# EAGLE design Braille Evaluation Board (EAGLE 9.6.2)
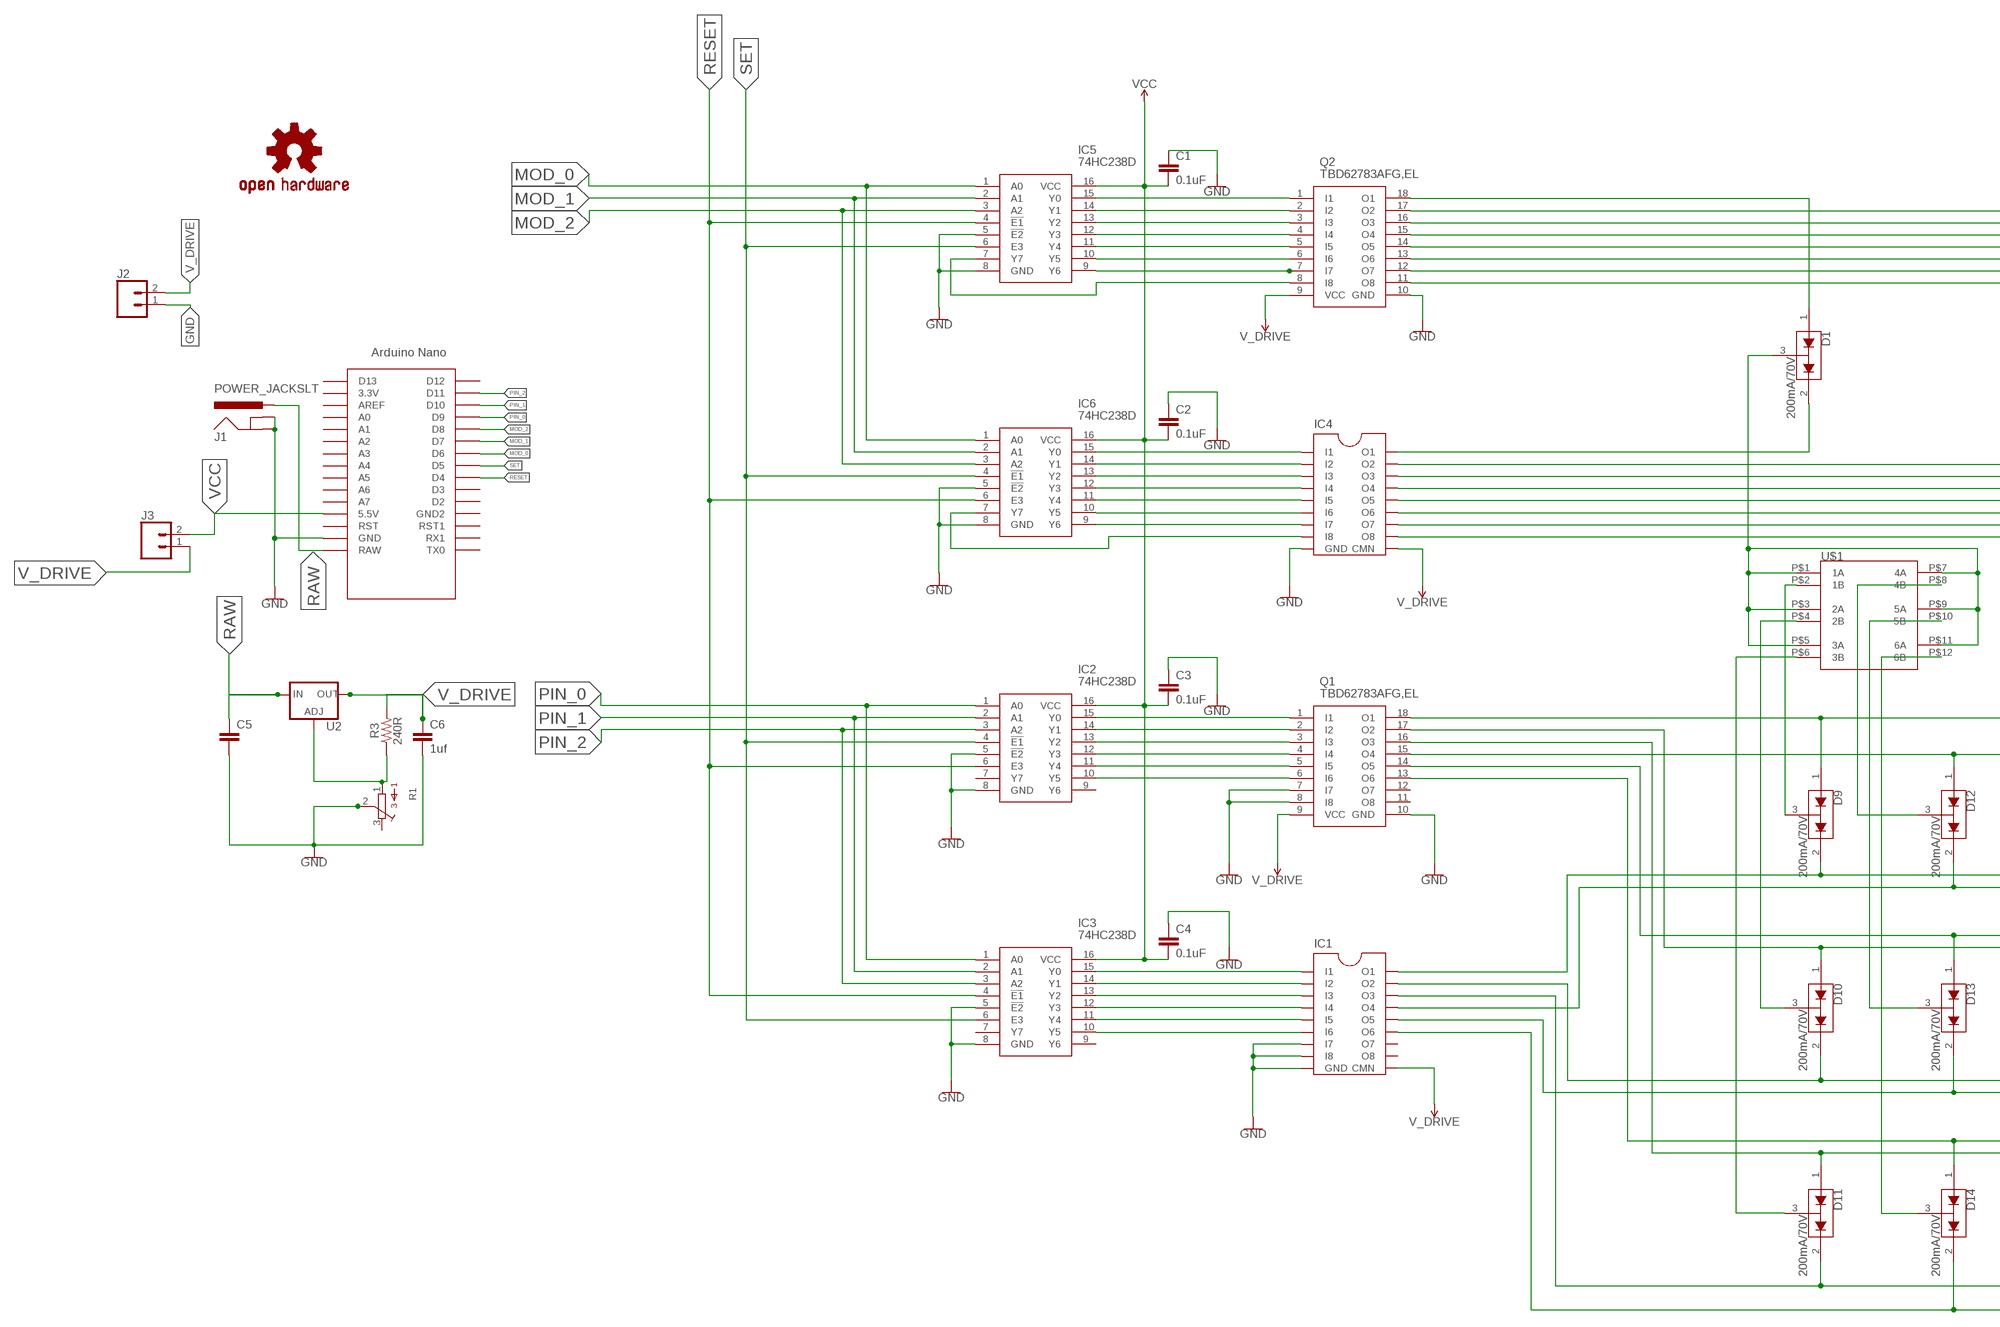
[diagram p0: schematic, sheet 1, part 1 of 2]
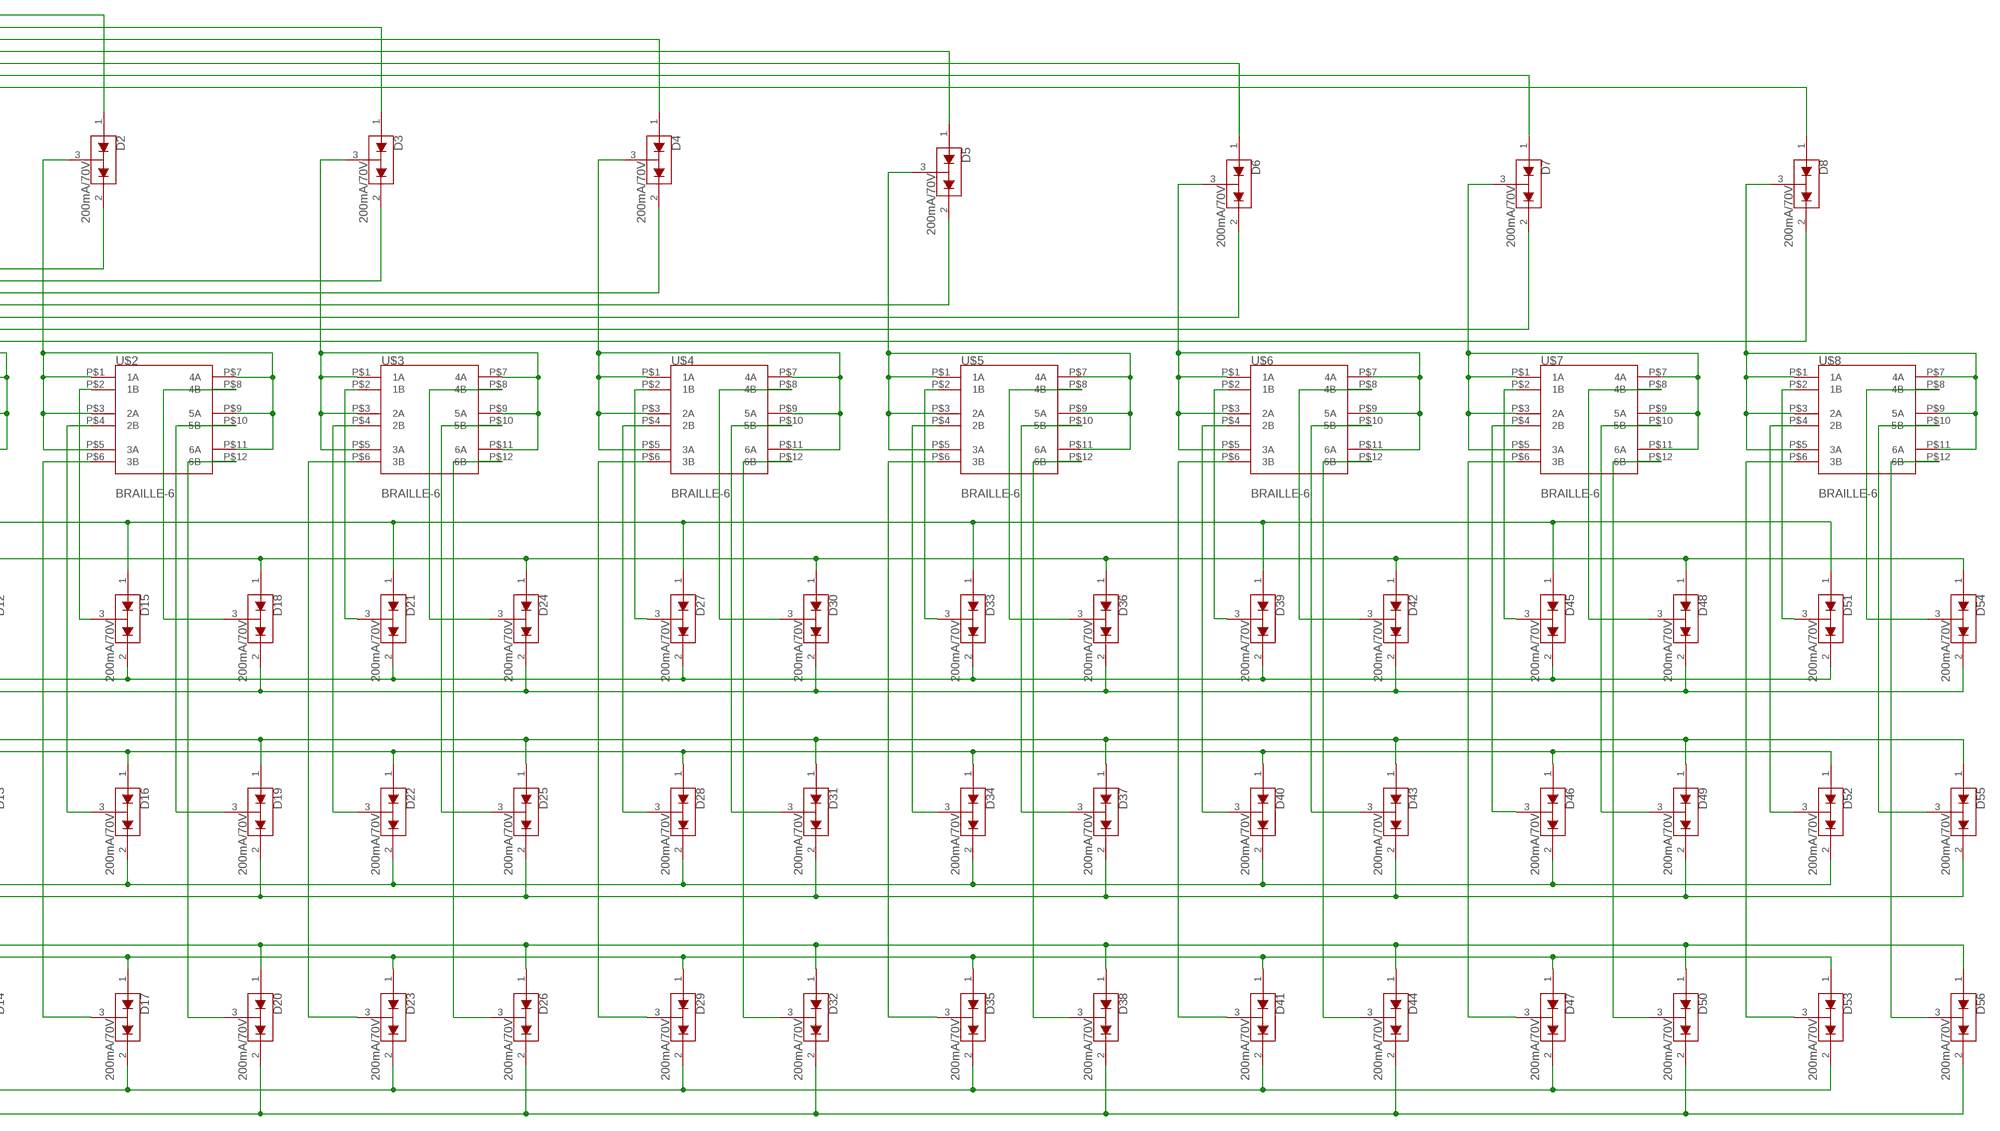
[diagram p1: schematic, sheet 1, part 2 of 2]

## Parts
C1  0.1uF  0.1UF-0603-25V-(+80/-20%)  [0603]
C2  0.1uF  0.1UF-0603-25V-(+80/-20%)  [0603]
C3  0.1uF  0.1UF-0603-25V-(+80/-20%)  [0603]
C4  0.1uF  0.1UF-0603-25V-(+80/-20%)  [0603]
C5  0.1uF  9.0PF-0603-50V-10%  [0603]
C6  1uf  9.0PF-0603-50V-10%  [0603]
D1  200mA/70V  BAV99  [SOT23-3]
D2  200mA/70V  BAV99  [SOT23-3]
D3  200mA/70V  BAV99  [SOT23-3]
D4  200mA/70V  BAV99  [SOT23-3]
D5  200mA/70V  BAV99  [SOT23-3]
D6  200mA/70V  BAV99  [SOT23-3]
D7  200mA/70V  BAV99  [SOT23-3]
D8  200mA/70V  BAV99  [SOT23-3]
D9  200mA/70V  BAV99  [SOT23-3]
D10  200mA/70V  BAV99  [SOT23-3]
D11  200mA/70V  BAV99  [SOT23-3]
D12  200mA/70V  BAV99  [SOT23-3]
D13  200mA/70V  BAV99  [SOT23-3]
D14  200mA/70V  BAV99  [SOT23-3]
D15  200mA/70V  BAV99  [SOT23-3]
D16  200mA/70V  BAV99  [SOT23-3]
D17  200mA/70V  BAV99  [SOT23-3]
D18  200mA/70V  BAV99  [SOT23-3]
D19  200mA/70V  BAV99  [SOT23-3]
D20  200mA/70V  BAV99  [SOT23-3]
D21  200mA/70V  BAV99  [SOT23-3]
D22  200mA/70V  BAV99  [SOT23-3]
D23  200mA/70V  BAV99  [SOT23-3]
D24  200mA/70V  BAV99  [SOT23-3]
D25  200mA/70V  BAV99  [SOT23-3]
D26  200mA/70V  BAV99  [SOT23-3]
D27  200mA/70V  BAV99  [SOT23-3]
D28  200mA/70V  BAV99  [SOT23-3]
D29  200mA/70V  BAV99  [SOT23-3]
D30  200mA/70V  BAV99  [SOT23-3]
D31  200mA/70V  BAV99  [SOT23-3]
D32  200mA/70V  BAV99  [SOT23-3]
D33  200mA/70V  BAV99  [SOT23-3]
D34  200mA/70V  BAV99  [SOT23-3]
D35  200mA/70V  BAV99  [SOT23-3]
D36  200mA/70V  BAV99  [SOT23-3]
D37  200mA/70V  BAV99  [SOT23-3]
D38  200mA/70V  BAV99  [SOT23-3]
D39  200mA/70V  BAV99  [SOT23-3]
D40  200mA/70V  BAV99  [SOT23-3]
D41  200mA/70V  BAV99  [SOT23-3]
D42  200mA/70V  BAV99  [SOT23-3]
D43  200mA/70V  BAV99  [SOT23-3]
D44  200mA/70V  BAV99  [SOT23-3]
D45  200mA/70V  BAV99  [SOT23-3]
D46  200mA/70V  BAV99  [SOT23-3]
D47  200mA/70V  BAV99  [SOT23-3]
D48  200mA/70V  BAV99  [SOT23-3]
D49  200mA/70V  BAV99  [SOT23-3]
D50  200mA/70V  BAV99  [SOT23-3]
D51  200mA/70V  BAV99  [SOT23-3]
D52  200mA/70V  BAV99  [SOT23-3]
D53  200mA/70V  BAV99  [SOT23-3]
D54  200mA/70V  BAV99  [SOT23-3]
D55  200mA/70V  BAV99  [SOT23-3]
D56  200mA/70V  BAV99  [SOT23-3]
IC1  TD62083  [SO18]
IC2  74HC238D  [SOIC127P600X175-16N]
IC3  74HC238D  [SOIC127P600X175-16N]
IC4  TD62083  [SO18]
IC5  74HC238D  [SOIC127P600X175-16N]
IC6  74HC238D  [SOIC127P600X175-16N]
J1  POWER_JACKSLT  [POWER_JACK_SLOT]
J2  CONN_02  [1X02]
J3  CONN_02  [1X02]
LOGO1  OSHW-LOGOL-COPPER  [OSHW-LOGO-L_COPPER]
Q1  TBD62783AFG,EL  [SOIC127P1030X245-18N]
Q2  TBD62783AFG,EL  [SOIC127P1030X245-18N]
R1  3362P  [3362P]
R3  240R  RESISTOR0603  [0603]
U2  LM317  V_REG_317SMD  [SOT223]
U$1  BRAILLE-6  [BRAILLE-6]
U$2  BRAILLE-6  [BRAILLE-6]
U$3  BRAILLE-6  [BRAILLE-6]
U$4  BRAILLE-6  [BRAILLE-6]
U$5  BRAILLE-6  [BRAILLE-6]
U$6  BRAILLE-6  [BRAILLE-6]
U$7  BRAILLE-6  [BRAILLE-6]
U$8  BRAILLE-6  [BRAILLE-6]
U$9  NANO  [NANO]

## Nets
GND: C1.1 C2.1 C3.1 C4.1 C5.2 C6.2 IC1.7(I7) IC1.8(I8) IC1.9(GND) IC2.5(!E2) IC2.8(GND) IC3.5(!E2) IC3.8(GND) IC4.9(GND) IC5.5(!E2) IC5.8(GND) IC6.5(!E2) IC6.8(GND) J1.GND@1(GNDBREAK) J1.GND@2(GND) J2.1 Q1.7(I7) Q1.8(I8) Q1.10(GND) Q2.10(GND) R1.2 U$9.GND
MOD_0: IC5.1(A0) IC6.1(A0) U$9.D6
MOD_1: IC5.2(A1) IC6.2(A1) U$9.D7
MOD_2: IC5.3(A2) IC6.3(A2) U$9.D8
N$1: IC2.15(Y0) Q1.1(I1)
N$2: IC2.14(Y1) Q1.2(I2)
N$3: IC2.13(Y2) Q1.3(I3)
N$4: IC2.12(Y3) Q1.4(I4)
N$5: IC2.11(Y4) Q1.5(I5)
N$6: IC2.10(Y5) Q1.6(I6)
N$7: IC1.1(I1) IC3.15(Y0)
N$8: IC1.2(I2) IC3.14(Y1)
N$9: IC1.3(I3) IC3.13(Y2)
N$10: IC1.4(I4) IC3.12(Y3)
N$11: IC1.5(I5) IC3.11(Y4)
N$12: IC5.15(Y0) Q2.1(I1)
N$13: IC5.14(Y1) Q2.2(I2)
N$14: IC5.13(Y2) Q2.3(I3)
N$15: IC5.12(Y3) Q2.4(I4)
N$16: IC5.11(Y4) Q2.5(I5)
N$17: D1.1(A1) Q2.18(O1)
N$18: IC4.1(I1) IC6.15(Y0)
N$19: IC4.2(I2) IC6.14(Y1)
N$20: IC4.3(I3) IC6.13(Y2)
N$21: IC4.4(I4) IC6.12(Y3)
N$22: IC4.5(I5) IC6.11(Y4)
N$23: D2.1(A1) Q2.17(O2)
N$24: IC5.10(Y5) Q2.6(I6)
N$25: D3.1(A1) Q2.16(O3)
N$26: IC5.9(Y6) Q2.7(I7)
N$27: IC5.7(Y7) Q2.8(I8)
N$28: IC4.8(I8) IC6.7(Y7)
N$29: IC4.6(I6) IC6.10(Y5)
N$30: IC4.7(I7) IC6.9(Y6)
N$31: D4.1(A1) Q2.15(O4)
N$32: IC1.6(I6) IC3.10(Y5)
N$33: D5.1(A1) Q2.14(O5)
N$34: D6.1(A1) Q2.13(O6)
N$35: D7.1(A1) Q2.12(O7)
N$36: D8.1(A1) Q2.11(O8)
N$37: D1.2(C2) IC4.18(O1)
N$38: D9.3(COM) U$1.P$2(1B)
N$39: D2.2(C2) IC4.17(O2)
N$40: D3.3(COM) U$3.P$1(1A) U$3.P$3(2A) U$3.P$5(3A) U$3.P$7(4A) U$3.P$9(5A) U$3.P$11(6A)
N$41: D4.3(COM) U$4.P$1(1A) U$4.P$3(2A) U$4.P$5(3A) U$4.P$7(4A) U$4.P$9(5A) U$4.P$11(6A)
N$42: D5.3(COM) U$5.P$1(1A) U$5.P$3(2A) U$5.P$5(3A) U$5.P$7(4A) U$5.P$9(5A) U$5.P$11(6A)
N$43: D6.3(COM) U$6.P$1(1A) U$6.P$3(2A) U$6.P$5(3A) U$6.P$7(4A) U$6.P$9(5A) U$6.P$11(6A)
N$44: D7.3(COM) U$7.P$1(1A) U$7.P$3(2A) U$7.P$5(3A) U$7.P$7(4A) U$7.P$9(5A) U$7.P$11(6A)
N$45: D8.3(COM) U$8.P$1(1A) U$8.P$3(2A) U$8.P$5(3A) U$8.P$7(4A) U$8.P$9(5A) U$8.P$11(6A)
N$46: D10.3(COM) U$1.P$4(2B)
N$47: D11.3(COM) U$1.P$6(3B)
N$48: D12.3(COM) U$1.P$8(4B)
N$49: D13.3(COM) U$1.P$10(5B)
N$50: D14.3(COM) U$1.P$12(6B)
N$51: D21.3(COM) U$3.P$2(1B)
N$52: D10.1(A1) D16.1(A1) D22.1(A1) D28.1(A1) D34.1(A1) D40.1(A1) D46.1(A1) D52.1(A1) Q1.17(O2)
N$53: D11.1(A1) D17.1(A1) D23.1(A1) D29.1(A1) D35.1(A1) D41.1(A1) D47.1(A1) D53.1(A1) Q1.16(O3)
N$54: D12.1(A1) D18.1(A1) D24.1(A1) D30.1(A1) D36.1(A1) D42.1(A1) D48.1(A1) D54.1(A1) Q1.15(O4)
N$55: D27.3(COM) U$4.P$2(1B)
N$56: D33.3(COM) U$5.P$2(1B)
N$57: D9.2(C2) D15.2(C2) D21.2(C2) D27.2(C2) D33.2(C2) D39.2(C2) D45.2(C2) D51.2(C2) IC1.18(O1)
N$58: D39.3(COM) U$6.P$2(1B)
N$59: D11.2(C2) D17.2(C2) D23.2(C2) D29.2(C2) D35.2(C2) D41.2(C2) D47.2(C2) D53.2(C2) IC1.16(O3)
N$60: D12.2(C2) D18.2(C2) D24.2(C2) D30.2(C2) D36.2(C2) D42.2(C2) D48.2(C2) D54.2(C2) IC1.15(O4)
N$61: D13.2(C2) D19.2(C2) D25.2(C2) D31.2(C2) D37.2(C2) D43.2(C2) D49.2(C2) D55.2(C2) IC1.14(O5)
N$62: D14.2(C2) D20.2(C2) D26.2(C2) D32.2(C2) D38.2(C2) D44.2(C2) D50.2(C2) D56.2(C2) IC1.13(O6)
N$63: D15.3(COM) U$2.P$2(1B)
N$64: D16.3(COM) U$2.P$4(2B)
N$65: D17.3(COM) U$2.P$6(3B)
N$66: D18.3(COM) U$2.P$8(4B)
N$67: D19.3(COM) U$2.P$10(5B)
N$68: D20.3(COM) U$2.P$12(6B)
N$69: D28.3(COM) U$4.P$4(2B)
N$70: D22.3(COM) U$3.P$4(2B)
N$71: D23.3(COM) U$3.P$6(3B)
N$72: D24.3(COM) U$3.P$8(4B)
N$73: D25.3(COM) U$3.P$10(5B)
N$74: D26.3(COM) U$3.P$12(6B)
N$75: D45.3(COM) U$7.P$2(1B)
N$76: D10.2(C2) D16.2(C2) D22.2(C2) D28.2(C2) D34.2(C2) D40.2(C2) D46.2(C2) D52.2(C2) IC1.17(O2)
N$77: D51.3(COM) U$8.P$2(1B)
N$78: D1.3(COM) U$1.P$1(1A) U$1.P$3(2A) U$1.P$5(3A) U$1.P$7(4A) U$1.P$9(5A) U$1.P$11(6A)
N$79: D2.3(COM) U$2.P$1(1A) U$2.P$3(2A) U$2.P$5(3A) U$2.P$7(4A) U$2.P$9(5A) U$2.P$11(6A)
N$80: D29.3(COM) U$4.P$6(3B)
N$81: D30.3(COM) U$4.P$8(4B)
N$82: D3.2(C2) IC4.16(O3)
N$83: D13.1(A1) D19.1(A1) D25.1(A1) D31.1(A1) D37.1(A1) D43.1(A1) D49.1(A1) D55.1(A1) Q1.14(O5)
N$84: D14.1(A1) D20.1(A1) D26.1(A1) D32.1(A1) D38.1(A1) D44.1(A1) D50.1(A1) D56.1(A1) Q1.13(O6)
N$85: D4.2(C2) IC4.15(O4)
N$86: D5.2(C2) IC4.14(O5)
N$87: D6.2(C2) IC4.13(O6)
N$88: D7.2(C2) IC4.12(O7)
N$89: D8.2(C2) IC4.11(O8)
N$91: D31.3(COM) U$4.P$10(5B)
N$92: D32.3(COM) U$4.P$12(6B)
N$93: R1.1 R3.1 U2.1(ADJ)
N$103: D34.3(COM) U$5.P$4(2B)
N$104: D35.3(COM) U$5.P$6(3B)
N$105: D36.3(COM) U$5.P$8(4B)
N$106: D37.3(COM) U$5.P$10(5B)
N$107: D38.3(COM) U$5.P$12(6B)
N$118: D40.3(COM) U$6.P$4(2B)
N$119: D41.3(COM) U$6.P$6(3B)
N$120: D42.3(COM) U$6.P$8(4B)
N$121: D43.3(COM) U$6.P$10(5B)
N$122: D44.3(COM) U$6.P$12(6B)
N$133: D46.3(COM) U$7.P$4(2B)
N$134: D47.3(COM) U$7.P$6(3B)
N$135: D48.3(COM) U$7.P$8(4B)
N$136: D49.3(COM) U$7.P$10(5B)
N$137: D50.3(COM) U$7.P$12(6B)
N$148: D52.3(COM) U$8.P$4(2B)
N$149: D53.3(COM) U$8.P$6(3B)
N$150: D54.3(COM) U$8.P$8(4B)
N$151: D55.3(COM) U$8.P$10(5B)
N$152: D56.3(COM) U$8.P$12(6B)
N$153: D9.1(A1) D15.1(A1) D21.1(A1) D27.1(A1) D33.1(A1) D39.1(A1) D45.1(A1) D51.1(A1) Q1.18(O1)
PIN_0: IC2.1(A0) IC3.1(A0) U$9.D9
PIN_1: IC2.2(A1) IC3.2(A1) U$9.D10
PIN_2: IC2.3(A2) IC3.3(A2) U$9.D11
RAW: C5.1 J1.PWR U2.3(IN) U$9.RAW
RESET: IC2.6(E3) IC3.4(!E1) IC5.4(!E1) IC6.6(E3) U$9.D4
SET: IC2.4(!E1) IC3.6(E3) IC5.6(E3) IC6.4(!E1) U$9.D5
V_DRIVE: C6.1 IC1.10(CMN) IC4.10(CMN) J2.2 J3.1 Q1.9(VCC) Q2.9(VCC) R3.2 U2.2(OUT)
VCC: C1.2 C2.2 C3.2 C4.2 IC2.16(VCC) IC3.16(VCC) IC5.16(VCC) IC6.16(VCC) J3.2 U$9.5V(5.5V)
Unconnected: IC1.11(O8) IC1.12(O7) IC2.7(Y7) IC2.9(Y6) IC3.7(Y7) IC3.9(Y6) Q1.11(O8) Q1.12(O7) R1.3 U$9.3.3V U$9.A0 U$9.A1 U$9.A2 U$9.A3 U$9.A4 U$9.A5 U$9.A6 U$9.A7 U$9.AREF U$9.D2 U$9.D3 U$9.D12 U$9.D13 U$9.GND1(GND2) U$9.ICSP1 U$9.ICSP2 U$9.ICSP3 U$9.ICSP4 U$9.ICSP5 U$9.ICSP6 U$9.RST U$9.RST1 U$9.RX1 U$9.TX0

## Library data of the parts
C1-C4 = SparkFun-Capacitors:0.1UF: 0.1µF ceramic capacitors; PROD_ID: CAP-00810
C5 C6 = SparkFun-Capacitors:9.0PF: 9.0pF ceramic capacitors; PROD_ID: CAP-09341; VALUE: 9.0pF
D1-D56 = SparkFun-DiscreteSemi:BAV99: Series-pair diode array Two small signal silicon diodes connected anode to cathode. Connections to all three nodes available. Link to datasheet SparkFun Products: SparkFun AutoDriver; PROD_ID: DIO-10647
IC1 IC4 = toshiba-td62083:TD62083: 8ch Darlington Sink Driver Source: http://akizukidenshi.com/download/TD62083AP.pdf
IC2 IC3 IC5 IC6 = 74HC238D:74HC238D: Codeurs, dcodeurs, multiplexeurs et dmultiplexeurs 3-TO-8 DECODER DEMULTIPLEXER Source: Datasheet; DESCRIPTION: Codeurs, dcodeurs, multiplexeurs et dmultiplexeurs 3-TO-8 DECODER DEMULTIPLEXER; HEIGHT: 1.75mm; MANUFACTURER_NAME: Nexperia; MANUFACTURER_PART_NUMBER: 74HC238D; MOUSER_PART_NUMBER: 771-74HC238D; MOUSER_PRICE-STOCK: https://www.mouser.co.uk/ProductDetail/Nexperia/74HC238D?qs=JTOGeJziEKGZLH3gr9jJBw%3D%3D
J1 = SparkFun-Connectors:POWER_JACK: Power Jack Connector This is the standard 5.5mm barrel jack for power. The PTH is the most common, proven, reliable, footprint. The Slot footprint only works if the mill layer is transmitted to the PCB fab house so be warned. Here are the connectors we sell at SparkFun: DC Barrel Power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; PROD_ID: PRT-00119
J2 J3 = SparkFun-Connectors:CONN_02: Multi connection point. Often used as Generic Header-pin footprint for 0.1 inch spaced/style header connections
LOGO1 = SparkFun-Aesthetics:OSHW-LOGO: Open-Source Hardware (OSHW) Logo
Q1 Q2 = TBD62783AFG_EL:TBD62783AFG,EL: Gate Drivers DMOS Transistor Array8-CH, 50V/0.5A Source: Datasheet; DESCRIPTION: Gate Drivers DMOS Transistor Array8-CH, 50V/0.5A; HEIGHT: 2.45mm; MANUFACTURER_NAME: Toshiba; MANUFACTURER_PART_NUMBER: TBD62783AFG,EL; MOUSER_PART_NUMBER: 757-TBD62783AFGEL; MOUSER_PRICE-STOCK: https://www.mouser.co.uk/ProductDetail/Toshiba/TBD62783AFGEL?qs=fSnNYG2PaKJyPGRf9HI0JA%3D%3D
R1 = bourns:3362: 3362 Series 1/4" Square Trimmer
R3 = SparkFun-Resistors:RESISTOR: Generic Resistor Package
U2 = SparkFun-IC-Power:V_REG_317: Voltage Regulator Standard LM317 adjustable voltage regulator. AOI (Adjust Output Input). Google 'LM317 Calculator' for easy to use app to get the two resistor values needed. 240/720 for 5V output. 240/390 for 3.3V output. Spark Fun Electronics SKU : COM-00527
U$1-U$8 = Braille Cell:BRAILLE-6
U$9 = Arduino-clone:NANO: Arduino Nano

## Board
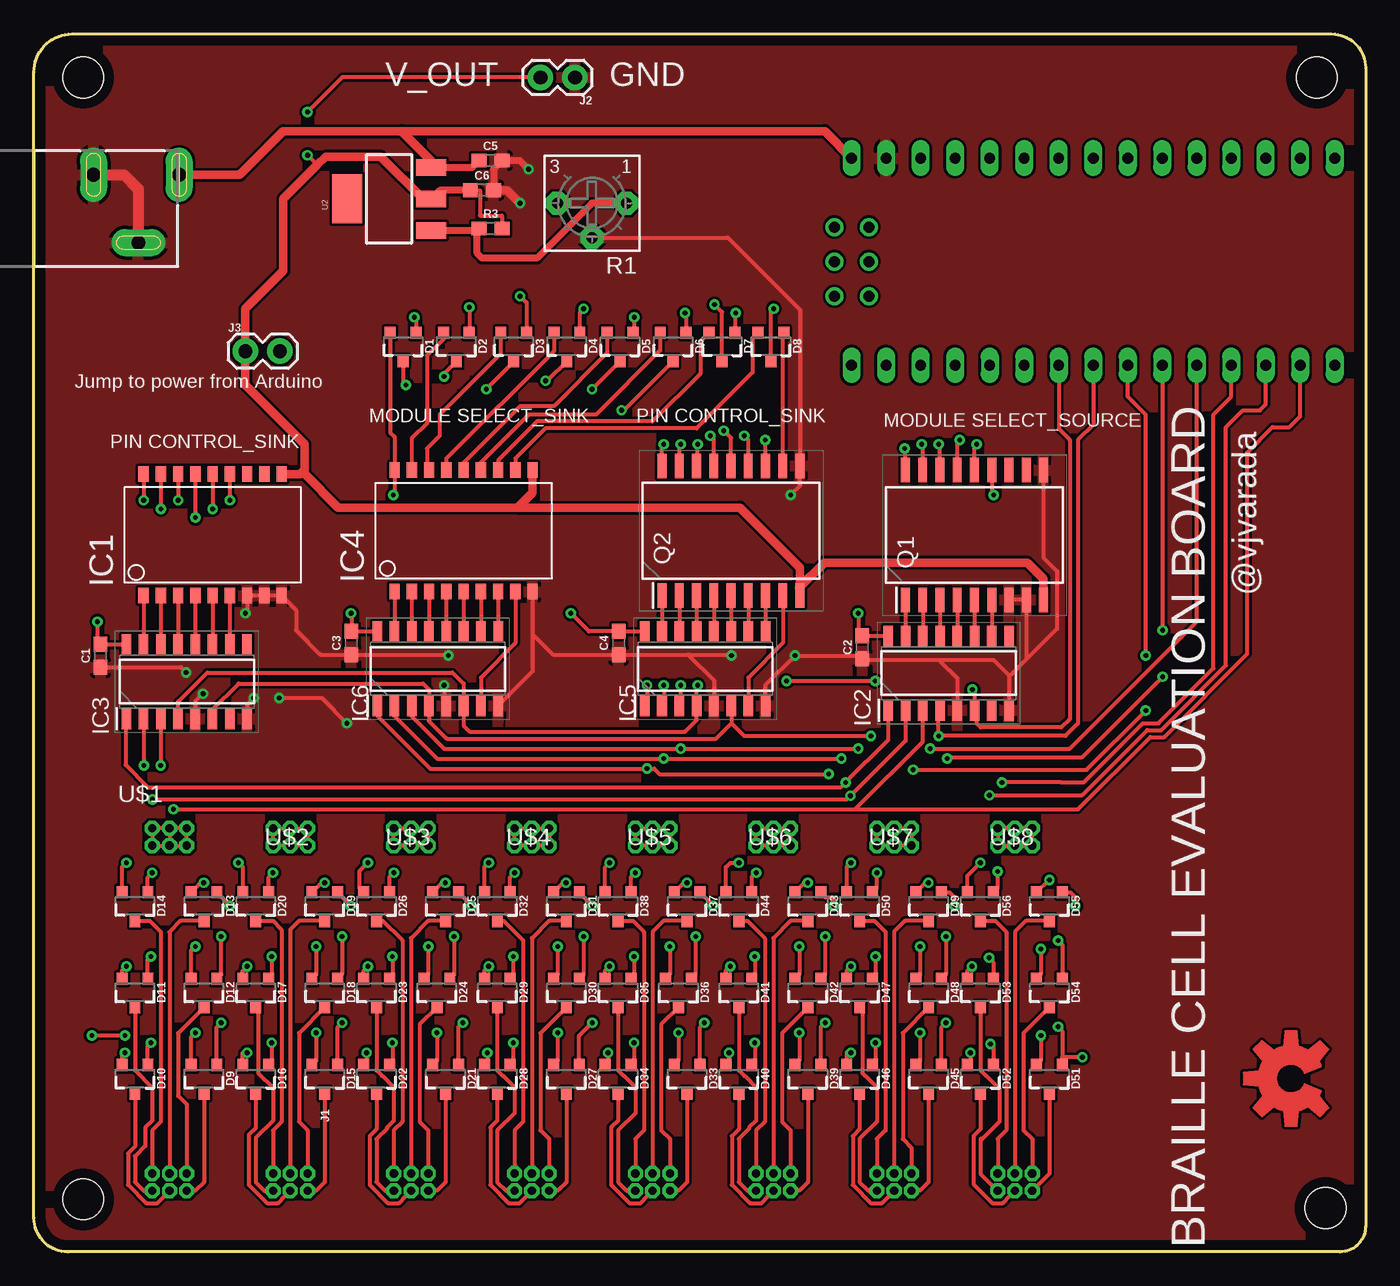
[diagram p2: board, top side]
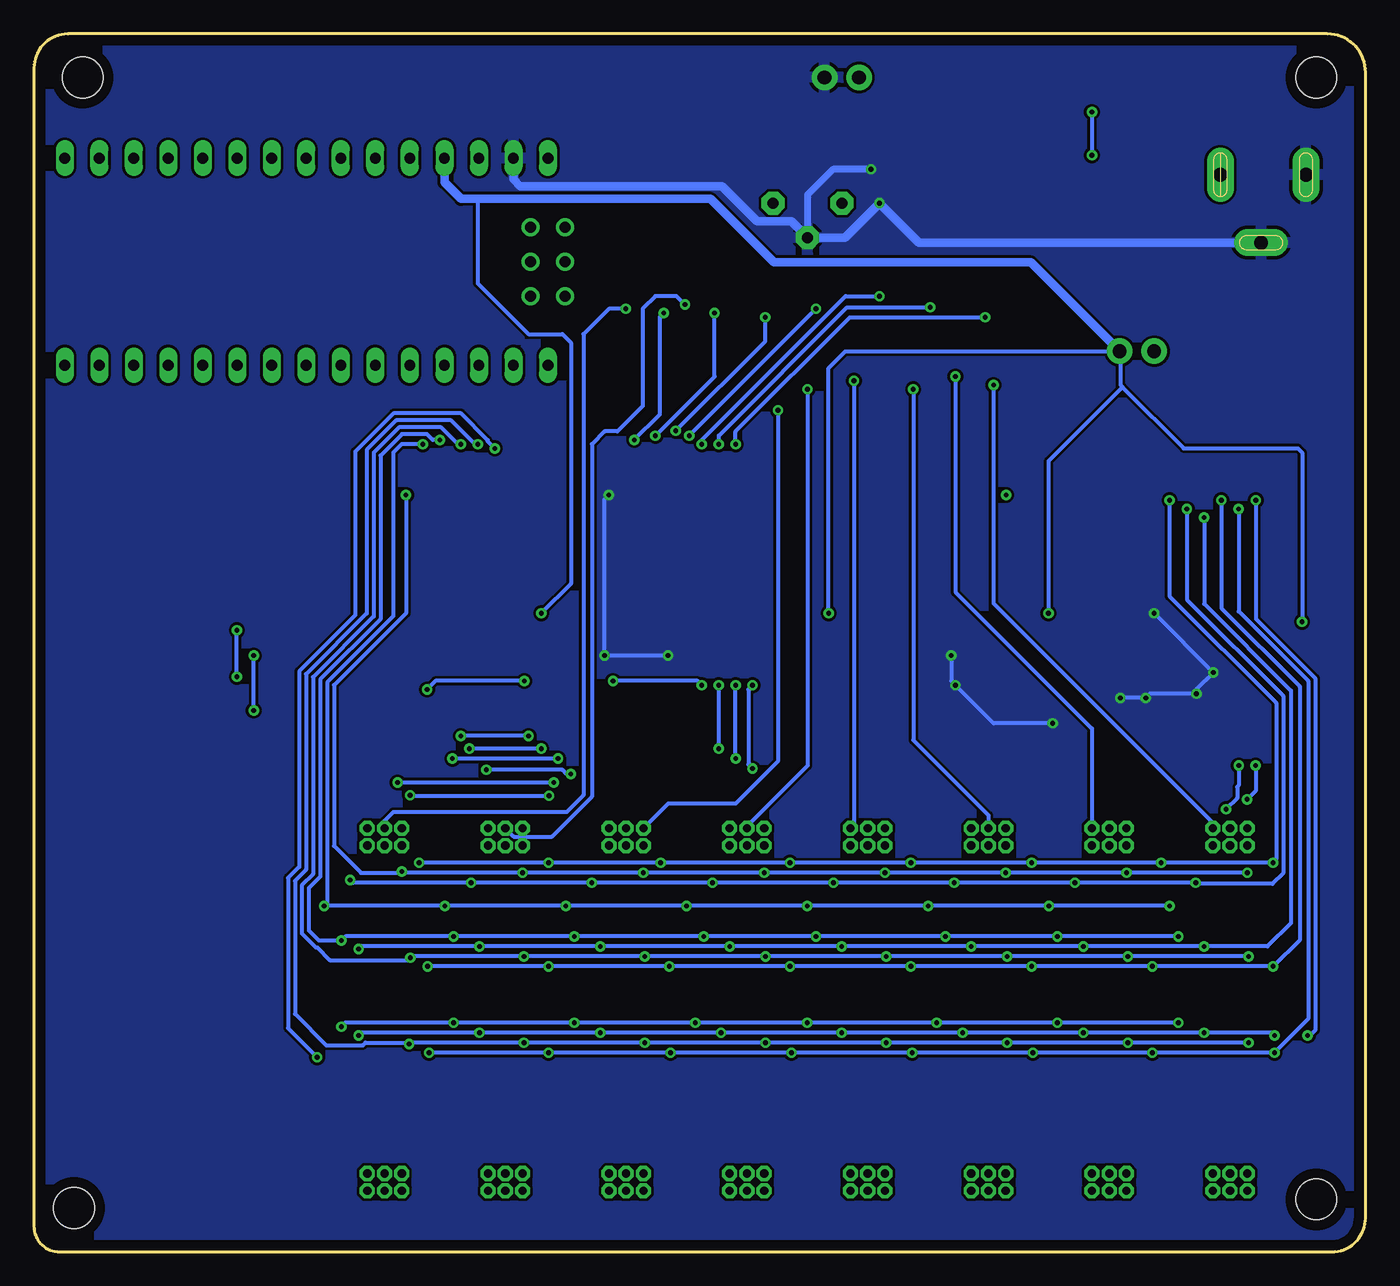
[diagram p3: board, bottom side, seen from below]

Size 98.01 x 89.61 mm. Coordinates in mm from the lower left corner, seen from the top.
Outline: 2.8,89.61 95.52,89.61 arc-90 98.01,87.12 98.01,1.87 arc-90 96.15,0 2.49,0 arc-90 0,2.49 0,86.81 arc-90 2.8,89.61
Copper layers (1*16): Top 0.035mm / dielectric 1.5mm / Bottom 0.035mm
Design rules "LionCircuits": minimum track width 8mil, minimum drill 0.35mm, track to track 8mil, track to pad 8mil, pad to pad 8mil, via to via 8mil, smd to smd 8mil, copper to edge 30mil, drill to drill 10mil, minimum pad ring 10mil, minimum via ring 8mil, stop-mask expansion 4mil, vias tented up to drill 0mil, thermal gap 10mil
Holes 3 mm at 3.63,86.41 3.63,3.86 95.07,3.23 94.43,86.41

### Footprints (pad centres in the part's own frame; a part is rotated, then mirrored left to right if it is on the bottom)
0603 = smd 1.1 x 1: 1 -0.85,0; 2 0.85,0
SOT23-3 = smd 0.8 x 0.9: 1 -0.95,-1; 2 0.95,-1; 3 0,1.1
SO18 = smd 0.762 x 1.143: 1 -5.08,-3.835; 2 -3.81,-3.835; 3 -2.54,-3.835; 4 -1.27,-3.835; 5 0,-3.835; 6 1.27,-3.835; 7 2.54,-3.835; 8 3.81,-3.835; 9 5.08,-3.835; 10 5.08,5.105; 11 3.81,5.105; 12 2.54,5.105; 13 1.27,5.105; 14 0,5.105; 15 -1.27,5.105; 16 -2.54,5.105; 17 -3.81,5.105; 18 -5.08,5.105
SOIC127P600X175-16N = smd 1.55 x 0.7: 1 -2.725,4.445; 2 -2.725,3.175; 3 -2.725,1.905; 4 -2.725,0.635; 5 -2.725,-0.635; 6 -2.725,-1.905; 7 -2.725,-3.175; 8 -2.725,-4.445; 9 2.725,-4.445; 10 2.725,-3.175; 11 2.725,-1.905; 12 2.725,-0.635; 13 2.725,0.635; 14 2.725,1.905; 15 2.725,3.175; 16 2.725,4.445
POWER_JACK_SLOT = drill 1 pad 2 long: GND@1 2.58,7.5; GND@2 7.58,10.8; PWR 2.58,13.8
1X02 = drill 1.016 pad 1.88: 1 0,0; 2 2.54,0
SOIC127P1030X245-18N = smd 1.8 x 0.65: 1 -4.775,5.08; 2 -4.775,3.81; 3 -4.775,2.54; 4 -4.775,1.27; 5 -4.775,0; 6 -4.775,-1.27; 7 -4.775,-2.54; 8 -4.775,-3.81; 9 -4.775,-5.08; 10 4.775,-5.08; 11 4.775,-3.81; 12 4.775,-2.54; 13 4.775,-1.27; 14 4.775,0; 15 4.775,1.27; 16 4.775,2.54; 17 4.775,3.81; 18 4.775,5.08
3362P = drill 0.813 pad 1.676 octagon: 1 -2.54,0; 2 0,2.54; 3 2.54,0
SOT223 = smd 1.219 x 2.235: 1 -2.311,-3.099; 2 0,-3.099; 3 2.311,-3.099 | smd 3.6 x 2.2: 4 0,3.099
BRAILLE-6 = drill 0.6 octagon: P$1 -1.27,13.335; P$2 1.27,-13.335; P$3 0,13.335; P$4 0,-13.335; P$5 1.27,13.335; P$6 -1.27,-13.335; P$7 -1.27,12.065; P$8 1.27,-12.065; P$9 0,12.065; P$10 0,-12.065; P$11 1.27,12.065; P$12 -1.27,-12.065
NANO = drill 0.8 long: 3.3V -10.16,24.13; 5V -10.16,-1.27; A0 -10.16,19.05; A1 -10.16,16.51; A2 -10.16,13.97; A3 -10.16,11.43; A4 -10.16,8.89; A5 -10.16,6.35; A6 -10.16,3.81; A7 -10.16,1.27; AREF -10.16,21.59; D2 5.08,1.27; D3 5.08,3.81; D4 5.08,6.35; D5 5.08,8.89; D6 5.08,11.43; D7 5.08,13.97; D8 5.08,16.51; D9 5.08,19.05; D10 5.08,21.59; D11 5.08,24.13; D12 5.08,26.67; D13 -10.16,26.67; GND -10.16,-6.35; GND1 5.08,-1.27; RAW -10.16,-8.89; RST -10.16,-3.81; RST1 5.08,-3.81; RX1 5.08,-6.35; TX0 5.08,-8.89 | drill 0.8: ICSP1 -5.08,-10.16; ICSP2 -5.08,-7.62; ICSP3 -2.54,-10.16; ICSP4 -2.54,-7.62; ICSP5 0,-10.16; ICSP6 0,-7.62

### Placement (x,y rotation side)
C1  4.9,43.87 90 top
C2  60.97,44.49 90 top
C3  23.36,44.8 90 top
C4  43.04,44.8 90 top
C5  33.6,80.29 0 top
C6  32.97,78.11 0 top
D1  27.18,66.64 180 top
D2  31.09,66.64 180 top
D3  35.31,66.64 180 top
D4  39.22,66.64 180 top
D5  43.14,66.64 180 top
D6  47.05,66.64 180 top
D7  50.65,66.64 180 top
D8  54.25,66.64 180 top
D9  12.52,12.75 180 top
D10  7.44,12.75 180 top
D11  7.44,19.1 180 top
D12  12.52,19.1 180 top
D13  12.52,25.45 180 top
D14  7.44,25.45 180 top
D15  21.41,12.75 180 top
D16  16.33,12.75 180 top
D17  16.33,19.1 180 top
D18  21.41,19.1 180 top
D19  21.41,25.45 180 top
D20  16.33,25.45 180 top
D21  30.3,12.75 180 top
D22  25.22,12.75 180 top
D23  25.22,19.1 180 top
D24  29.66,19.1 180 top
D25  30.3,25.45 180 top
D26  25.22,25.45 180 top
D27  39.19,12.75 180 top
D28  34.11,12.75 180 top
D29  34.11,19.1 180 top
D30  39.19,19.1 180 top
D31  39.19,25.45 180 top
D32  34.11,25.45 180 top
D33  48.08,12.75 180 top
D34  43,12.75 180 top
D35  43,19.1 180 top
D36  47.44,19.1 180 top
D37  48.08,25.45 180 top
D38  43,25.45 180 top
D39  56.97,12.75 180 top
D40  51.89,12.75 180 top
D41  51.89,19.1 180 top
D42  56.97,19.1 180 top
D43  56.97,25.45 180 top
D44  51.89,25.45 180 top
D45  65.86,12.75 180 top
D46  60.78,12.75 180 top
D47  60.78,19.1 180 top
D48  65.86,19.1 180 top
D49  65.86,25.45 180 top
D50  60.78,25.45 180 top
D51  74.75,12.75 180 top
D52  69.67,12.75 180 top
D53  69.67,19.1 180 top
D54  74.75,19.1 180 top
D55  74.75,25.45 180 top
D56  69.67,25.45 180 top
IC1  13.15,52.12 0 top
IC2  67.32,42.58 90 top
IC3  11.25,41.96 90 top
IC4  31.62,52.42 0 top
IC5  49.4,42.89 90 top
IC6  29.72,42.89 90 top
J1  -3.11,81.83 270 top
J2  39.82,86.41 180 top
J3  15.56,66.27 0 top
LOGO1  92.53,12.75 90 top
Q1  69.23,52.74 90 top
Q2  51.31,53.05 90 top
R1  41.07,77.17 180 top
R3  33.6,75.3 0 top
U2  26.14,77.48 90 top
U$1  9.98,17.83 0 top
U$2  18.87,17.83 0 top
U$3  27.76,17.83 0 top
U$4  36.65,17.83 0 top
U$5  45.54,17.83 0 top
U$6  54.43,17.83 0 top
U$7  63.32,17.83 0 top
U$8  72.21,17.83 0 top
U$9  69.08,70.32 270 top

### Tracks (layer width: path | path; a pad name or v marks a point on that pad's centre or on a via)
GND  (via drill 0.35)
  Top 0.305: 66.59,43.56 61.05,43.56 C2.1 60.74,43.87 v56.01,43.87 53.85,41.71 IC5.8 | 66.59,43.56 67.96,42.19 IC2.5 | 66.59,43.56 70.63,43.56 71.77,42.42 71.77,42.32 | 71.77,42.32 IC2.8 | 73.04,43.59 Q1.8 Q1.7 | 73.04,43.59 71.77,42.32 | 48.15,43.95 C4.1 38.19,43.95 36.72,45.43 | IC5.5 50.04,42.06 48.15,43.95 | IC4.9 36.72,45.43 | 36.72,45.43 36.72,42.72 IC6.8 | v30.49,43.87 30.42,43.95 C3.1 21.08,43.95 19.29,45.74 19.29,47.22 IC1.9 IC1.8 IC1.7 15.69,47.12 v15.56,46.98 | v30.18,41.69 30.18,40.34 IC6.5 | C1.1 10.81,43.02 v11.2,42.63 | v12.45,41.07 11.88,40.51 IC3.5 | v16.18,40.76 15.69,40.27 IC3.8 | v18.05,40.76 21.16,40.76 v23.02,38.89 | 48.15,43.95 51.26,43.95 v51.34,43.87 | 74.31,56.88 Q1.10 74.31,51.09 75.3,50.09 75.3,45.85 73.04,43.59 | v55.7,55.7 56.39,56.39 Q2.10 56.39,69.32 51.08,74.62 R1.2
  Top 0.508: C6.2 33.82,79.65 C5.2 35.77,80.29 v36.4,79.65 | J1.GND@2 7.69,75.89 | 5.69,79.25 J1.GND@1
  Top 0.61: C6.2 34.84,78.11 v35.78,77.16
  Top 0.813: J1.GND@1 6.62,79.25 7.69,78.19 J1.GND@2
  Bottom 0.305: v30.49,43.87 30.49,42 v30.18,41.69 27.38,38.89 v23.02,38.89 | v15.56,46.98 v11.2,42.63 12.45,41.38 v12.45,41.07 15.87,41.07 v16.18,40.76 v18.05,40.76 | v51.34,43.87 v56.01,43.87 56.01,55.38 v55.7,55.7
  Bottom 0.508: v36.4,79.65 39.2,79.65 41.07,77.79 R1.2
  Bottom 0.61: J1.GND@2 32.87,74.25 v35.78,77.16 38.32,74.62 R1.2 42.27,75.82 44.79,75.82 47.38,78.41 62.23,78.41 62.72,78.9 U$9.GND
  pour Top: -0.18,90.22 98.24,90.22 98.24,-0.58 -0.18,-0.58
  pour Bottom: -0.18,90.22 98.24,90.22 98.24,-0.58 -0.18,-0.58
MOD_0  (via drill 0.35)
  Top 0.305: IC6.1 25.27,39.45 29.16,35.56 v45.12,35.56 45.65,35.56 46.05,35.16 v58.5,35.16 | v45.12,41.69 45.12,40.33 IC5.1 | v81.83,39.83 77.48,35.47 v64.72,35.47 | v81.83,43.87 81.83,61.61 80.5,62.93 U$9.D6
  Bottom 0.305: v45.12,35.56 45.43,35.87 45.43,41.38 v45.12,41.69 | v58.5,35.16 58.81,35.16 59.12,35.47 v64.72,35.47 | v81.83,39.83 v81.83,43.87
MOD_1  (via drill 0.35)
  Top 0.305: IC6.2 26.54,39.42 29.67,36.29 v46.36,36.29 v59.43,36.29 | v46.36,41.69 46.36,40.3 IC5.2 | v67.21,36.29 67.21,36.4 77.16,36.4 v83.08,42.32 | v83.08,45.74 83.08,65.21 U$9.D7
  Bottom 0.305: v46.36,36.29 v46.36,41.69 | v59.43,36.29 v67.21,36.29 | v83.08,42.32 v83.08,45.74
MOD_2  (via drill 0.35)
  Top 0.305: IC6.3 27.81,39.4 30.18,37.03 v47.61,37.03 v60.67,37.03 | v47.61,41.69 47.61,40.28 IC5.3 | v65.96,37.03 76.23,37.03 85.58,46.38 U$9.D8
  Bottom 0.305: v47.61,37.03 v47.61,41.69 | v60.67,37.03 v65.96,37.03
N$1
  Top 0.305: Q1.1 IC2.15
N$2
  Top 0.305: Q1.2 IC2.14
N$3
  Top 0.305: Q1.3 IC2.13
N$4
  Top 0.305: Q1.4 IC2.12
N$5
  Top 0.305: Q1.5 IC2.11
N$6
  Top 0.305: Q1.6 IC2.10
N$7
  Top 0.305: IC1.1 IC3.15
N$8
  Top 0.305: IC1.2 IC3.14
N$9
  Top 0.305: IC1.3 IC3.13
N$10
  Top 0.305: IC1.4 IC3.12
N$11
  Top 0.305: IC1.5 IC3.11
N$12
  Top 0.305: Q2.1 IC5.15
N$13
  Top 0.305: Q2.2 IC5.14
N$14
  Top 0.305: Q2.3 IC5.13
N$15
  Top 0.305: Q2.4 IC5.12
N$16
  Top 0.305: Q2.5 IC5.11
N$17  (via drill 0.35)
  Top 0.305: Q2.18 46.23,59.3 v46.36,59.43 | v28,68.76 28.13,68.64 D1.1
  Bottom 0.305: v28,68.76 37.96,68.76 46.36,60.36 v46.36,59.43
N$18
  Top 0.305: IC4.1 IC6.15
N$19
  Top 0.305: IC4.2 IC6.14
N$20
  Top 0.305: IC4.3 IC6.13
N$21
  Top 0.305: IC4.4 IC6.12
N$22
  Top 0.305: IC4.5 IC6.11
N$23  (via drill 0.35)
  Top 0.305: Q2.17 47.5,59.32 v47.61,59.43 | v32.05,69.5 32.05,67.65 D2.1
  Bottom 0.305: v47.61,59.43 47.61,60.05 38.16,69.5 v32.05,69.5
N$24
  Top 0.305: Q2.6 IC5.10
N$25  (via drill 0.35)
  Top 0.305: Q2.16 48.85,57.91 v48.85,59.43 | v35.78,70.32 36.26,69.84 D3.1
  Bottom 0.305: v48.85,59.43 48.85,59.74 38.27,70.32 v35.78,70.32
N$26
  Top 0.305: Q2.7 IC5.9
N$27
  Top 0.305: Q2.8 55.12,44.8 52.58,42.26 IC5.7
N$28
  Top 0.305: IC4.8 35.43,44.8 32.89,42.26 IC6.7
N$29
  Top 0.305: IC4.6 IC6.10
N$30
  Top 0.305: IC4.7 IC6.9
N$31  (via drill 0.35)
  Top 0.305: Q2.15 50.04,59.8 v49.78,60.05 | v40.45,69.39 40.17,69.11 D4.1
  Bottom 0.305: v49.78,60.05 v40.45,69.39
N$32
  Top 0.305: IC1.6 IC3.10
N$33  (via drill 0.35)
  Top 0.305: Q2.14 51.31,59.88 v50.77,60.42 | v44.18,68.76 44.18,67.73 D5.1
  Bottom 0.305: v50.77,60.42 44.18,67.01 v44.18,68.76
N$34  (via drill 0.35)
  Top 0.305: Q2.13 52.58,59.75 v52.27,60.05 | v47.92,69.07 48,68.99 D6.1
  Bottom 0.305: v52.27,60.05 47.92,64.41 v47.92,69.07
N$35  (via drill 0.35)
  Top 0.305: Q2.12 53.83,57.85 v53.83,59.74 | v51.65,69.07 51.6,69.02 D7.1
  Bottom 0.305: v53.83,59.74 51.96,61.61 51.96,68.76 v51.65,69.07
N$36
  Top 0.305: Q2.11 55.12,67.56 D8.1
N$37  (via drill 0.35)
  Top 0.305: v26.45,55.7 26.54,55.79 IC4.18 26.54,59.96 26.23,60.27 D1.2
N$38
  Top 0.305: D9.3 12.52,5.13 11.88,4.5 U$1.P$2
N$39
  Top 0.305: D2.2 30.14,67.17 28.94,65.96 28.94,60.99 27.81,59.86 IC4.17
N$40  (via drill 0.35)
  Top 0.305: U$3.P$3 U$3.P$1 U$3.P$7 U$3.P$9 | U$3.P$3 U$3.P$5 U$3.P$11 | U$3.P$11 U$3.P$9 | U$3.P$3 U$3.P$9 | U$3.P$11 29.2,30.07 | D3.3 35.31,65.49 v33.29,63.47
  Bottom 0.305: v33.29,63.47 33.29,37.65 27.76,32.11 U$3.P$3
N$41  (via drill 0.35)
  Top 0.305: U$4.P$3 U$4.P$1 U$4.P$7 U$4.P$9 | U$4.P$3 U$4.P$5 U$4.P$11 U$4.P$9 | U$4.P$3 U$4.P$9 | D4.3 37.78,64.1 v37.65,64.1
  Bottom 0.305: v37.65,64.1 37.65,31.43 U$4.P$5
N$42  (via drill 0.35)
  Top 0.305: U$5.P$3 U$5.P$1 U$5.P$7 U$5.P$9 | U$5.P$3 U$5.P$5 U$5.P$11 | U$5.P$11 U$5.P$9 | U$5.P$3 U$5.P$9 | U$5.P$11 46.98,30.07 | D5.3 v41.07,63.47
  Bottom 0.305: v41.07,63.47 41.07,35.78 45.54,31.32 U$5.P$3
N$43  (via drill 0.35)
  Top 0.305: U$6.P$11 U$6.P$5 U$6.P$3 U$6.P$1 U$6.P$7 U$6.P$9 U$6.P$11 | U$6.P$11 55.87,30.07 | D6.3 43.43,61.92 v43.25,61.92
  Bottom 0.305: v43.25,61.92 43.25,36.09 46.36,32.98 51.34,32.98 U$6.P$1
N$44  (via drill 0.35)
  Top 0.305: U$7.P$11 U$7.P$5 U$7.P$3 U$7.P$1 U$7.P$7 U$7.P$9 U$7.P$11 | U$7.P$11 64.76,30.07 | D7.3 50.65,69.14 v50.09,69.7
  Bottom 0.305: v50.09,69.7 50.72,70.32 52.27,70.32 53.21,69.39 53.21,62.23 55.07,60.36 56.01,60.36 56.94,59.43 56.94,33.5 59.89,30.54 62.69,30.54 U$7.P$3
N$45  (via drill 0.35)
  Top 0.305: U$8.P$11 U$8.P$9 U$8.P$7 U$8.P$1 U$8.P$3 U$8.P$5 U$8.P$11 | U$8.P$11 73.65,30.07 | D8.3 54.25,69.18 v54.45,69.39
  Bottom 0.305: v54.45,69.39 55.7,69.39 57.56,67.52 57.56,33.6 58.81,32.36 71.56,32.36 72.21,31.72 U$8.P$3
N$46
  Top 0.305: D10.3 7.44,7.75 6.93,7.25 6.93,4.92 8.26,3.59 9.08,3.59 9.62,4.12 9.62,4.14 U$1.P$4
N$47
  Top 0.305: D11.3 7.44,13.35 8.71,12.08 8.71,9.66 8.2,9.15 8.2,7.8 7.44,7.04 7.44,5.13 8.07,4.5 U$1.P$6
N$48
  Top 0.305: D12.3 10.61,16.1 10.61,11.48 11.25,10.85 U$1.P$8
N$49
  Top 0.305: U$1.P$10 9.98,23.55 10.78,24.35 D13.3
N$50
  Top 0.305: D14.3 8.54,24.35 9.34,23.55 9.34,9.58 8.71,8.94 U$1.P$12
N$51
  Top 0.305: D21.3 30.3,5.13 29.66,4.5 U$3.P$2
N$52  (via drill 0.35)
  Top 0.305: D10.1 8.39,15.17 v8.61,15.39 | v70.4,15.29 70.62,15.07 D52.1 | v61.95,15.39 61.95,13.97 D46.1 | v53.06,15.39 53.06,13.97 D40.1 | v44.17,15.39 44.17,13.97 D34.1 | v26.39,15.39 26.39,13.97 D22.1 | v35.28,15.39 35.28,13.97 D28.1 | v17.5,15.39 17.5,13.97 D16.1 | Q1.17 65.42,59.35 v65.34,59.43
  Bottom 0.305: v8.61,15.39 v17.5,15.39 v26.39,15.39 | 26.49,15.29 v26.39,15.39 | v26.39,15.39 v35.28,15.39 v44.17,15.39 v53.06,15.39 v61.95,15.39 70.3,15.39 | 70.3,15.39 v70.4,15.29 | v65.34,59.43 65.55,59.43 67.3,61.18 71.35,61.18 73.51,59.01 73.51,46.97 77.98,42.5 77.98,28.12 78.8,27.3 78.8,17.51 76.49,15.19 73.81,15.19 73.61,15.39 70.3,15.39
N$53  (via drill 0.35)
  Top 0.305: D11.1 8.39,21.52 v8.61,21.74 | v70.3,21.64 70.62,21.33 D53.1 | v61.95,21.74 61.95,20.32 D47.1 | v53.06,21.74 53.06,20.32 D41.1 | v44.17,21.74 44.17,20.32 D35.1 | v35.28,21.74 35.28,20.32 D29.1 | v26.39,21.74 26.39,20.32 D23.1 | v17.5,21.74 17.5,20.32 D17.1 | Q1.16 66.69,59.33 v66.59,59.43
  Bottom 0.305: v8.61,21.74 v17.5,21.74 v26.39,21.74 v35.28,21.74 v44.17,21.74 v53.06,21.74 v61.95,21.74 70.2,21.74 v70.3,21.64 70.47,21.47 76.23,21.47 77.16,22.4 77.26,22.4 78.3,23.44 78.3,26.97 77.48,27.79 77.48,42.29 73.01,46.76 73.01,58.8 71.14,60.67 68.03,60.67 66.79,59.43 v66.59,59.43
N$54  (via drill 0.35)
  Top 0.305: D12.1 13.79,20.42 v13.79,23.21 | v75.38,22.91 75.7,22.6 D54.1 | v67.13,23.21 67.13,20.42 D48.1 | v58.24,23.21 58.24,20.42 D42.1 | v48.71,23.21 48.71,20.42 D36.1 | v40.46,23.21 40.46,20.42 D30.1 | v30.93,23.21 30.93,20.42 D24.1 | v22.68,23.21 22.68,20.42 D18.1 | Q1.15 67.96,59.56 v68.14,59.74
  Bottom 0.305: v13.79,23.21 v22.68,23.21 v30.93,23.21 v40.46,23.21 v48.71,23.21 v58.24,23.21 v67.13,23.21 75.08,23.21 v75.38,22.91 77.05,22.91 77.79,23.65 77.79,26.76 76.94,27.61 76.94,42.11 72.5,46.55 72.5,58.59 70.93,60.16 69.08,60.16 68.66,59.74 v68.14,59.74
N$55
  Top 0.305: D27.3 39.19,5.13 38.55,4.5 U$4.P$2
N$56
  Top 0.305: D33.3 48.08,5.13 47.44,4.5 U$5.P$2
N$57  (via drill 0.35)
  Top 0.305: D9.2 11.57,15.81 v11.88,16.12 | v74.11,15.93 74.11,14.07 D51.2 | v65.22,16.12 65.22,14.07 D45.2 | v56.33,16.12 56.33,14.07 D39.2 | v47.44,16.12 47.44,14.07 D33.2 | v38.55,16.12 38.55,14.07 D27.2 | v29.66,16.12 29.66,14.07 D21.2 | v20.77,16.12 20.77,14.07 D15.2 | IC1.18 v8.07,55.3 | v4.26,15.93 v6.7,15.93
  Bottom 0.305: v74.11,15.93 73.91,16.12 v65.22,16.12 v56.33,16.12 v47.44,16.12 v38.55,16.12 v29.66,16.12 v20.77,16.12 v11.88,16.12 6.9,16.12 v6.7,15.93 | v4.26,15.93 4.08,15.93 3.71,16.29 3.71,42.22 8.07,46.57 v8.07,55.3
N$58
  Top 0.305: D39.3 56.97,5.13 56.33,4.5 U$6.P$2
N$59  (via drill 0.35)
  Top 0.305: D11.2 6.49,20.69 v6.8,21.01 | D17.2 15.38,20.69 v15.69,21.01 | D23.2 24.27,20.69 v24.58,21.01 | D29.2 33.16,20.69 v33.47,21.01 | D35.2 42.05,20.69 v42.36,21.01 | D41.2 50.94,20.69 v51.25,21.01 | D47.2 59.83,20.69 v60.14,21.01 | D53.2 68.72,20.69 v69.03,21.01 | IC1.16 v10.61,55.3
  Bottom 0.305: v69.03,21.01 v60.14,21.01 v51.25,21.01 v42.36,21.01 v33.47,21.01 v24.58,21.01 v15.69,21.01 v6.8,21.01 6.78,21.01 4.86,22.92 4.86,41.61 10.61,47.36 v10.61,55.3
N$60  (via drill 0.35)
  Top 0.305: D12.2 11.57,22.16 v11.88,22.47 | D54.2 74.11,20.42 v74.11,22.28 | v65.22,22.47 65.22,20.42 D48.2 | v56.33,22.47 56.33,20.42 D42.2 | v46.81,22.47 46.81,20.42 D36.2 | v38.55,22.47 38.55,20.42 D30.2 | v29.03,22.47 29.03,20.42 D24.2 | v20.77,22.47 20.77,20.42 D18.2 | IC1.15 v11.88,54.03
  Bottom 0.305: v74.11,22.28 73.91,22.47 v65.22,22.47 v56.33,22.47 v46.81,22.47 v38.55,22.47 v29.03,22.47 v20.77,22.47 v11.88,22.47 7.21,22.47 5.49,24.19 5.49,41.29 11.88,47.68 v11.88,54.03
N$61  (via drill 0.35)
  Top 0.305: D13.2 12.27,27.16 v12.5,27.16 | D19.2 21.16,27.16 v21.39,27.16 | D25.2 30.05,27.16 v30.28,27.16 | D37.2 47.83,27.16 v48.06,27.16 | D43.2 56.72,27.16 v56.95,27.16 | D31.2 38.94,27.16 v39.17,27.16 | D49.2 65.61,27.16 v65.84,27.16 | D55.2 74.7,27.36 v74.75,27.36 | IC1.14 v13.15,54.66
  Bottom 0.305: v74.75,27.36 74.55,27.16 v65.84,27.16 v56.95,27.16 v48.06,27.16 v39.17,27.16 v30.28,27.16 v21.39,27.16 v12.5,27.16 12.41,27.07 6.84,27.07 6.07,27.85 6.07,40.92 13.15,48 v13.15,54.66
N$62  (via drill 0.35)
  Top 0.305: D14.2 6.49,28.31 v6.8,28.63 | v15.06,28.63 15.38,28.31 D20.2 | v24.58,28.63 23.95,27.99 23.95,26.77 D26.2 | D32.2 33.16,28.31 v33.47,28.63 | D38.2 42.05,28.31 v42.36,28.63 | D44.2 50.94,28.31 51.25,28.63 v51.89,28.63 | D50.2 59.83,28.31 v60.14,28.63 | D56.2 68.72,27.68 v69.67,28.63 | IC1.13 v14.42,55.3
  Bottom 0.305: v6.8,28.63 6.84,28.63 | 6.84,28.63 v15.06,28.63 v24.58,28.63 v33.47,28.63 v42.36,28.63 v51.89,28.63 v60.14,28.63 v69.67,28.63 | v14.42,55.3 14.43,55.28 14.43,48.25 6.58,40.4 6.58,28.89 6.84,28.63
N$63
  Top 0.305: D15.3 21.41,5.13 20.77,4.5 U$2.P$2
N$64
  Top 0.305: U$2.P$4 18.51,4.14 18.51,4.12 17.97,3.59 17.15,3.59 15.82,4.92 15.82,8.6 16.33,9.11 D16.3
N$65
  Top 0.305: D17.3 16.52,17.81 16.52,13.15 17.6,12.08 17.6,9.66 16.33,8.39 16.33,5.13 16.96,4.5 U$2.P$6
N$66
  Top 0.305: D18.3 19.5,16.1 19.5,9.58 20.14,8.94 U$2.P$8
N$67
  Top 0.305: D19.3 19.5,24.35 18.87,23.72 U$2.P$10
N$68
  Top 0.305: D20.3 17.6,24.35 18.23,23.72 18.23,9.58 17.6,8.94 U$2.P$12
N$69
  Top 0.305: D28.3 34.11,9.66 33.6,9.15 33.6,4.92 34.93,3.59 35.75,3.59 36.29,4.12 36.29,4.14 U$4.P$4
N$70
  Top 0.305: D22.3 25.22,9.02 24.71,8.52 24.71,4.92 26.04,3.59 26.86,3.59 27.4,4.12 27.4,4.14 U$3.P$4
N$71
  Top 0.305: D23.3 25.22,13.35 25.62,12.94 25.66,12.94 26.49,12.12 26.49,9.66 25.98,9.15 25.98,9.07 25.22,8.31 25.22,5.13 25.85,4.5 U$3.P$6
N$72
  Top 0.305: D24.3 28.39,16.73 28.39,9.58 29.03,8.94 U$3.P$8
N$73
  Top 0.305: D25.3 29.03,24.35 27.76,23.08 U$3.P$10
N$74
  Top 0.305: 25.22,24.18 D26.3 25.68,24.35 27.12,22.91 27.12,9.58 26.49,8.94 U$3.P$12
N$75
  Top 0.305: D45.3 65.86,5.13 65.22,4.5 U$7.P$2
N$76  (via drill 0.35)
  Top 0.305: D10.2 6.49,14.44 v6.7,14.66 | IC1.17 v9.34,54.66 | D46.2 59.83,14.66 v60.14,14.66 | v68.93,14.66 68.93,13.75 D52.2 | v51.15,14.66 51.15,13.75 D40.2 | v42.26,14.66 42.26,13.75 D34.2 | v33.37,14.66 33.37,13.75 D28.2 | v24.48,14.66 24.48,13.75 D22.2 | D16.2 15.38,14.66 v15.69,14.66
  Bottom 0.305: v68.93,14.66 v60.14,14.66 v51.15,14.66 v42.26,14.66 v33.37,14.66 v24.48,14.66 v15.69,14.66 v6.7,14.66 4.22,17.13 4.22,42.01 9.34,47.12 v9.34,54.66
N$77
  Top 0.305: U$8.P$2 73.84,4.86 73.85,4.86 74.75,5.75 D51.3
N$78  (via drill 0.35)
  Top 0.305: U$1.P$9 U$1.P$7 U$1.P$1 U$1.P$3 | U$1.P$9 U$1.P$11 U$1.P$5 U$1.P$3 | U$1.P$3 U$1.P$9 | D1.3 27.18,63.99 v27.38,63.79
  Bottom 0.305: v27.38,63.79 27.38,47.71 11.2,31.53 11.2,31.21 U$1.P$5
N$79  (via drill 0.35)
  Top 0.305: U$2.P$3 U$2.P$1 U$2.P$7 U$2.P$9 | U$2.P$3 U$2.P$5 U$2.P$11 | U$2.P$11 U$2.P$9 | U$2.P$3 U$2.P$9 | U$2.P$11 20.31,30.07 | D2.3 30.18,64.63 v30.18,64.41
  Bottom 0.305: v30.18,64.41 30.18,48.54 20.14,38.49 U$2.P$5
N$80
  Top 0.305: D29.3 34.11,13.35 34.51,12.94 34.55,12.94 35.38,12.12 35.38,10.21 34.11,8.94 34.11,5.13 34.74,4.5 U$4.P$6
N$81
  Top 0.305: D30.3 37.28,16.1 37.28,8.94 37.92,8.31 U$4.P$8
N$82
  Top 0.305: D3.2 34.36,66.1 29.87,61.61 29.87,60.05 28.94,59.12 28.94,57.67 IC4.16
N$83  (via drill 0.35)
  Top 0.305: D13.1 14.42,25.5 v14.42,25.45 | D55.1 76.29,26.45 76.65,26.09 v76.65,25.45 | D49.1 67.4,26.45 67.76,26.09 v67.76,25.45 | D43.1 58.28,26.09 58.87,26.09 v58.87,25.45 | D37.1 49.98,25.5 v49.98,25.45 | D31.1 41.09,25.5 v41.09,25.45 | D25.1 32.2,25.5 v32.2,25.45 | D19.1 23.31,25.5 v23.31,25.45 | Q1.14 69.23,59.27 v69.39,59.43
  Bottom 0.305: v14.42,25.45 v23.31,25.45 v32.2,25.45 v41.09,25.45 v49.98,25.45 v58.87,25.45 v67.76,25.45 v76.65,25.45 76.43,25.67 76.43,41.9 71.56,46.77 71.56,58.81 70.94,59.43 v69.39,59.43
N$84  (via drill 0.35)
  Top 0.305: D14.1 8.39,27.57 v8.71,27.89 | D38.1 43.95,27.57 v44.27,27.89 | D32.1 35.06,27.57 v35.38,27.89 | D26.1 26.17,27.57 v26.49,27.89 | D56.1 70.94,26.77 v70.94,27.99 | D50.1 62.05,26.77 v62.05,27.89 | D44.1 52.84,27.57 v53.16,27.89 | D20.1 17.28,27.57 v17.6,27.89 | Q1.13 70.5,55.83 v70.63,55.7
  Bottom 0.305: v8.71,27.89 v17.6,27.89 v26.49,27.89 v35.38,27.89 v44.27,27.89 v53.16,27.89 v62.05,27.89 70.84,27.89 | 70.84,27.89 v70.94,27.99 | v70.63,55.7 70.63,46.98 75.92,41.69 75.92,29.87 73.94,27.89 70.84,27.89
N$85
  Top 0.305: D4.2 38.27,66.28 30.35,58.36 IC4.15
N$86
  Top 0.305: D5.2 42.19,66.14 38.27,62.23 35.78,62.23 31.62,58.07 IC4.14
N$87
  Top 0.305: D6.2 46.1,66.32 41.38,61.61 36.4,61.61 32.89,58.1 IC4.13
N$88
  Top 0.305: D7.2 49.05,66.99 49.05,64.63 45.52,61.1 37.03,61.1 34.16,58.24 IC4.12
N$89
  Top 0.305: D8.2 52.9,67.23 52.9,64.72 48.77,60.59 37.65,60.59 35.43,58.38 IC4.11
N$91
  Top 0.305: D31.3 37.92,24.35 36.65,23.08 U$4.P$10
N$92
  Top 0.305: D32.3 34.57,24.35 36.01,22.91 36.01,9.58 35.38,8.94 U$4.P$12
N$93
  Top 0.508: U2.1 32.62,75.16 | 32.62,75.16 R3.1 | R1.1 41.07,77.16 37.03,73.12 32.98,73.12 32.62,73.48 32.62,75.16
N$103
  Top 0.305: D34.3 43,9.66 42.49,9.15 42.49,4.92 43.82,3.59 44.64,3.59 45.18,4.12 45.18,4.14 U$5.P$4
N$104
  Top 0.305: D35.3 43,13.35 43.4,12.94 43.44,12.94 44.27,12.12 44.27,10.21 43,8.94 43,5.13 43.63,4.5 U$5.P$6
N$105
  Top 0.305: D36.3 46.17,16.73 46.17,8.94 46.81,8.31 U$5.P$8
N$106
  Top 0.305: D37.3 46.34,24.35 45.54,23.55 U$5.P$10
N$107
  Top 0.305: D38.3 44.1,24.35 44.9,23.55 44.9,8.94 44.27,8.31 U$5.P$12
N$118
  Top 0.305: D40.3 51.89,9.02 51.38,8.52 51.38,4.92 52.71,3.59 53.53,3.59 54.07,4.12 54.07,4.14 U$6.P$4
N$119
  Top 0.305: D41.3 51.89,13.35 52.29,12.94 52.33,12.94 53.16,12.12 53.16,9.66 52.65,9.15 52.65,9.07 51.89,8.31 51.89,5.13 52.52,4.5 U$6.P$6
N$120
  Top 0.305: D42.3 55.06,16.1 55.06,9.58 55.7,8.94 U$6.P$8
N$121
  Top 0.305: 56.97,24.18 D43.3 55.7,24.35 54.43,23.08 U$6.P$10
N$122
  Top 0.305: D44.3 52.52,24.35 53.79,23.08 53.79,9.58 53.16,8.94 U$6.P$12
N$133
  Top 0.305: D46.3 60.78,9.02 60.27,8.52 60.27,4.92 61.6,3.59 62.42,3.59 62.96,4.12 62.96,4.14 U$7.P$4
N$134
  Top 0.305: D47.3 60.97,17.81 60.97,13.15 61.18,12.94 61.22,12.94 62.05,12.12 62.05,9.58 60.78,8.31 60.78,5.13 61.41,4.5 U$7.P$6
N$135
  Top 0.305: D48.3 63.95,16.1 63.95,8.31 64.59,7.67 U$7.P$8
N$136
  Top 0.305: D49.3 64.12,24.35 63.32,23.55 U$7.P$10
N$137
  Top 0.305: D50.3 61.88,24.35 62.68,23.55 62.68,8.94 62.05,8.31 U$7.P$12
N$148
  Top 0.305: U$8.P$4 71.85,4.14 71.85,4.12 71.31,3.59 70.56,3.59 69.16,4.99 69.16,8.52 69.67,9.02 D52.3
N$149
  Top 0.305: D53.3 69.67,13.35 70.07,12.94 70.11,12.94 71.06,11.99 71.06,9.58 69.79,8.31 69.67,8.31 69.67,5.75 70.56,4.86 70.58,4.86 U$8.P$6
N$150
  Top 0.305: D54.3 72.84,16.1 72.84,8.94 73.48,8.31 U$8.P$8
N$151
  Top 0.305: D55.3 73.01,24.35 72.21,23.55 U$8.P$10
N$152
  Top 0.305: U$8.P$12 70.94,8.31 71.57,8.94 71.57,23.55 70.77,24.35 D56.3
N$153  (via drill 0.35)
  Top 0.305: D9.1 13.47,16.54 v13.79,16.86 | v75.38,16.56 75.7,16.25 75.7,14.31 | 75.7,14.31 D51.1 | D45.1 66.81,16.54 v67.13,16.86 | D39.1 57.92,16.54 v58.24,16.86 | D33.1 49.03,16.54 v49.35,16.86 | D27.1 40.14,15.9 v41.09,16.86 | D21.1 31.25,16.54 v31.57,16.86 | D15.1 22.36,16.54 v22.68,16.86 | Q1.18 64.15,59.07 v64.1,59.12 | v77.16,14.31 75.7,14.31
  Bottom 0.305: v13.79,16.86 v22.68,16.86 v31.57,16.86 v41.09,16.86 v49.35,16.86 v58.24,16.86 v67.13,16.86 75.08,16.86 v75.38,16.56 | v64.1,59.12 64.61,59.63 64.61,59.73 66.56,61.69 71.56,61.69 74.36,58.88 74.36,46.84 78.49,42.71 78.49,28.33 79.31,27.51 79.31,16.46 v77.16,14.31
PIN_0  (via drill 0.35)
  Top 0.305: IC3.1 6.74,39.18 6.74,35.82 8.36,34.2 59.41,34.2 v59.74,34.54 62.88,37.67 IC2.1 | v71.25,34.54 75.61,34.54 77.26,34.54 81.62,38.89 82.77,38.89 86.81,42.94 86.81,61.61 88.12,62.92 U$9.D9
  Bottom 0.305: v71.25,34.54 v59.74,34.54
PIN_1  (via drill 0.35)
  Top 0.305: IC3.2 8.07,35.8 v8.09,35.78 | v8.71,33.29 59.84,33.29 v60.1,33.56 64.15,37.6 IC2.2 | U$9.D10 90.66,62.35 90.23,61.92 88.99,61.92 87.74,60.67 87.74,43.15 82.98,38.39 81.95,38.39 77.16,33.6 v70.32,33.6
  Bottom 0.305: v8.09,35.78 8.09,33.92 v8.71,33.29 | v60.1,33.56 70.27,33.56 v70.32,33.6
PIN_2  (via drill 0.35)
  Top 0.305: IC3.3 v9.34,35.79 v9.33,35.78 | v10.27,32.56 60.44,32.56 | IC2.3 65.42,37.53 60.44,32.56 | 60.44,32.56 75.92,32.56 76.03,32.56 76.84,32.56 82.16,37.88 83.19,37.88 89.3,43.99 89.3,58.81 91.17,60.67 92.41,60.67 93.2,61.47 U$9.D11
  Bottom 0.305: v9.33,35.78 9.33,34.33 9.45,34.22 9.45,33.38 v10.27,32.56
RAW
  Top 0.508: U2.3 32.25,79.79 C5.1
  Top 0.61: J1.PWR 15.16,79.25 18.36,82.45 27.07,82.45 | U2.3 29.24,80.29 27.07,82.45 | 27.07,82.45 58.21,82.45 U$9.RAW
RESET  (via drill 0.35)
  Top 0.305: IC3.4 10.61,40.48 12.76,42.63 30.8,42.63 31.62,41.81 IC6.6 31.62,38.7 32.05,38.27 47.92,38.27 48.77,39.12 IC5.4 48.77,41.61 v48.85,41.69 | v55.38,42 v61.92,42 | v69.07,41.38 69.23,41.23 IC2.6 69.39,39.7 69.39,38.89 69.7,38.58 75.61,38.58 76.23,39.2 76.23,59.74 75.42,60.55 U$9.D4
  Bottom 0.305: v48.85,41.69 49.16,42 v55.38,42 | v61.92,42 68.45,42 v69.07,41.38
SET  (via drill 0.35)
  Top 0.305: 51.34,38.89 50.21,37.76 30.38,37.76 29.08,39.06 IC6.4 29.08,41.35 28.63,41.81 15.05,41.81 13.15,39.91 IC3.6 | 51.34,38.89 51.34,40.14 IC5.6 | 51.34,38.89 52.27,37.96 v61.61,37.96 | IC2.4 66.59,39.76 v66.59,37.96 75.92,37.96 76.85,38.89 76.85,59.74 77.96,60.85 U$9.D5
  Bottom 0.305: v61.61,37.96 v66.59,37.96
V_DRIVE  (via drill 0.35)
  Top 0.305: 56.39,48.95 Q2.9 56.39,48.85 56.32,48.85 | C6.1 32.84,78.11 32.84,76.25 34.45,76.25 R3.2 | J2.2 22.68,86.41 v20.14,83.87 | v20.14,80.7 20.86,79.97
  Top 0.508: C6.1 29.87,78.11 U2.2
  Top 0.61: 19.91,57.56 19.58,57.23 IC1.10 | U2.2 28.63,77.48 25.51,80.59 21.47,80.59 20.86,79.97 18.36,77.48 18.36,72.19 15.56,69.39 J3.1 15.56,63.79 19.91,59.43 19.91,57.56 | IC4.10 36.7,55.85 35.61,54.76 | 19.91,57.56 19.91,57.25 22.4,54.76 35.61,54.76 | 35.61,54.76 51.96,54.76 56.39,50.34 56.39,48.95 | Q1.9 74.31,49.53 73.12,50.72 58.18,50.72 56.32,48.85
  Bottom 0.305: v20.14,83.87 v20.14,80.7
VCC  (via drill 0.35)
  Top 0.305: IC3.16 4.93,44.69 C1.2 4.67,44.94 v4.67,46.36 | IC2.16 62.85,45.34 C2.2 60.67,45.64 v60.67,46.98 | IC6.16 23.38,45.62 | 23.38,45.62 C3.2 | IC5.16 43.07,45.62 C4.2 40.85,45.65 v39.52,46.98 | v23.34,46.98 23.38,46.93 23.38,45.62
  Bottom 0.305: J3.2 18.07,66.25 | 18.07,66.25 18.05,66.22 18.05,63.79 17.89,63.63 | 17.89,63.63 13.38,59.12 4.98,59.12 4.67,58.81 v4.67,46.36 | 17.89,63.63 23.34,58.18 v23.34,46.98 | 65.34,77.48 65.34,71.25 61.61,67.52 59.12,67.52 58.5,66.9 58.5,49.16 v60.67,46.98 | v39.52,46.98 39.52,65.03 38.3,66.25 18.07,66.25
  Bottom 0.61: J3.2 24.63,72.81 43.56,72.81 48.23,77.48 65.34,77.48 66.59,77.48 67.8,78.7 U$9.5V

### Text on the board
tNames: V_OUT | GND | Jump to power from Arduino | BRAILLE CELL EVALUATION BOARD | MODULE SELECT_SINK | PIN CONTROL_SINK | MODULE SELECT_SOURCE | PIN CONTROL_SINK | @vjvarada

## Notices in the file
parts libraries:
SparkFun-PowerSymbols: Licensing: Creative Commons ShareAlike 4.0 International - https://creativecommons.org/licenses/by-sa/4.0
